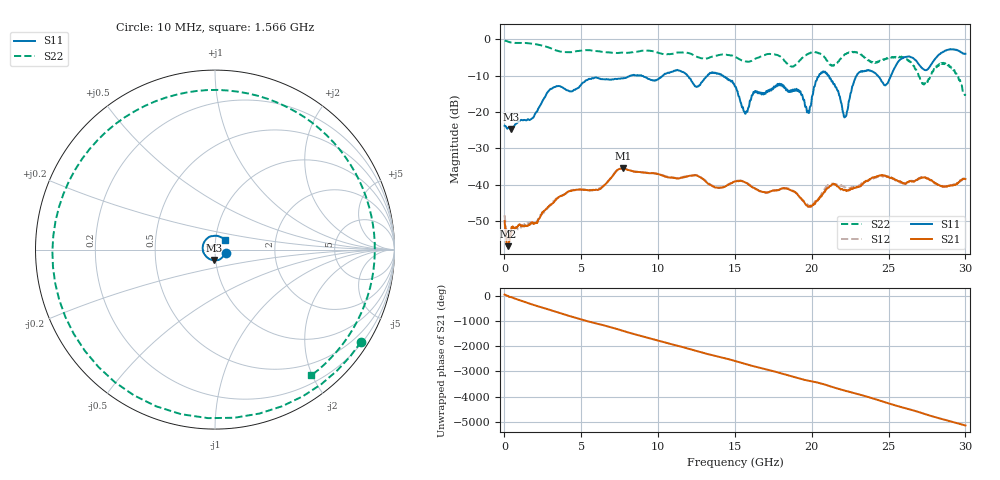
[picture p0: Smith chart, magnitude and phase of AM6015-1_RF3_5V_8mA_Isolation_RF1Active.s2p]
!Agilent Technologies,E8364B,MY43040894,A.07.50.67
!Agilent E8364B: A.07.50.67
!Date: Monday, August 13, 2018 07:05:40
!Correction: S11(Full 2 Port(1,2))
!S21(Full 2 Port(1,2))
!S12(Full 2 Port(1,2))
!S22(Full 2 Port(1,2))
!S2P File: Measurements: S11, S21, S12, S22:
# Hz S  dB  R 50
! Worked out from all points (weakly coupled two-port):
!   1601 points, 10 MHz to 30 GHz, reference 50 ohm
!   highest |S21| = -35.59 dB at 7.695 GHz (marker M1); lowest = -57.0 dB at 216.2 MHz (marker M2)
!   lowest |S11| = -24.7 dB at 403.6 MHz (marker M3), VSWR 1.12, Z = 49.2 - j5.75 ohm
!   |S11| at or under -10 dB: start of sweep to 8.232 GHz; 14.22 GHz to 20.47 GHz (6.251 GHz wide, 36 % of centre); 21.1 GHz to 22.93 GHz (1.821 GHz wide, 8.27 % of centre)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
!   |S22| runs from -15.4 to -0.3 dB; largest |S21 - S12| = 0.0049
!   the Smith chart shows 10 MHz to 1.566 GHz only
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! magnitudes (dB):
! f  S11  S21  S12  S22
! 10 MHz  -23.8  -50.1  -48.5  -0.3
! 216.2 MHz  -24.5  -57.0  -54.7  -0.6
! 403.6 MHz  -24.7  -53.8  -53.8  -0.9
! 3.084 GHz  -13.6  -45.4  -45.0  -2.6
! 5.015 GHz  -12.3  -41.5  -41.3  -3.1
! 7.695 GHz  -10.8  -35.6  -35.6  -3.7
! 10.02 GHz  -11.0  -37.2  -37.2  -3.8
! 13.62 GHz  -9.2  -40.6  -40.4  -4.7
! 15.01 GHz  -13.0  -39.2  -39.2  -4.9
! 15.7 GHz  -20.5  -39.5  -39.4  -6.1
! 16.24 GHz  -14.6  -40.9  -40.9  -5.5
! 17.89 GHz  -12.3  -41.4  -41.4  -4.6
! 19.71 GHz  -20.2  -45.8  -45.5  -4.1
! 20.01 GHz  -16.0  -45.9  -45.7  -3.6
! 20.87 GHz  -8.9  -41.8  -41.0  -5.1
! 22.17 GHz  -21.3  -41.6  -40.8  -4.1
! 23.08 GHz  -9.1  -40.6  -40.2  -3.9
! 25.01 GHz  -11.4  -38.0  -37.9  -5.0
! 26.08 GHz  -4.9  -39.8  -39.7  -5.2
! 27.3 GHz  -8.3  -38.1  -38.0  -12.5
! 28.8 GHz  -2.9  -40.6  -40.5  -6.8
! 30 GHz  -4.0  -38.5  -38.5  -15.2
